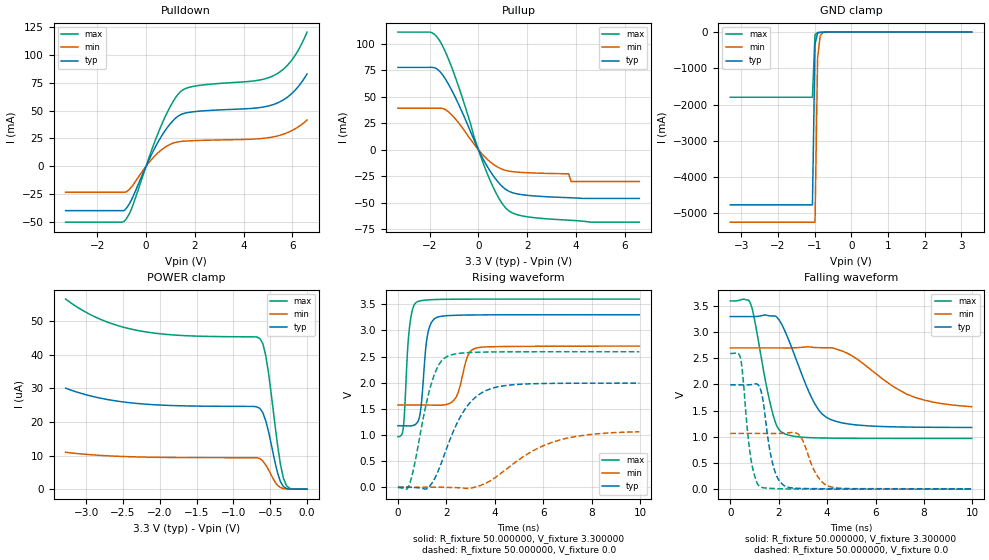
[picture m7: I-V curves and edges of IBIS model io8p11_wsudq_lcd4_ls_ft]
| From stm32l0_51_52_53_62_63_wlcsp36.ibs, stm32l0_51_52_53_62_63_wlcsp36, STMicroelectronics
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|   Model io8p11_wsudq_lcd4_ls_ft
[Model]  io8p11_wsudq_lcd4_ls_ft
Model_type I/O
Polarity   Non-Inverting
Enable   Active-Low
Vinl =   0.990000V
Vinh =   2.310000V
Vmeas =  1.650000V
Cref =   50.000000pF
Rref =   100.000000M
Vref =   0.0V
C_comp   3.263700pF   3.224800pF   3.309000pF
[Temperature Range]   25.000000   0.125000k   -40.000000
[Pullup Reference]   3.300000V   2.700000V   3.600000V
[Pulldown Reference]   0.0V   0.0V   0.0V
[POWER Clamp Reference]   3.300000V   2.700000V   3.600000V
[GND Clamp Reference]   0.0V   0.0V   0.0V
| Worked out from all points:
|   slope of the pulldown table from 0 to 0.495 V, typ, clamps not added: 22.6 ohm
|   slope of the pullup table from 0 to 0.495 V, typ, clamps not added: 23.9 ohm
|   GND clamp passes 1 mA (typ) near -0.64 V on its own axis
|   rising waveform, R_fixture 50.000000, V_fixture 3.300000: 20-80 % time 240ps typ, 378ps min, 202ps max; typ from 1.18 V to 3.3 V
|   rising waveform, R_fixture 50.000000, V_fixture 0.0: 20-80 % time 1.2ns typ, 2.22ns min, 722ps max; typ from 0 V to 1.99 V
|   falling waveform, R_fixture 50.000000, V_fixture 3.300000: 20-80 % time 1.14ns typ, 2.1ns min, 656ps max; typ from 3.3 V to 1.18 V
|   falling waveform, R_fixture 50.000000, V_fixture 0.0: 20-80 % time 417ps typ, 583ps min, 339ps max; typ from 1.99 V to 0 V
[Pulldown]
|Voltage   I(typ)   I(min)   I(max)
-3.3V     -39.83mA   -23.37mA   -50.2mA
-900mV    -39.83mA   -23.37mA   -49.52mA
-600mV    -30.28mA   -18.59mA   -38.45mA
500mV     22.11mA    12.28mA    30.1mA
1V        38.33mA    19.81mA    53.88mA
1.4V      46.1mA     22.18mA    66.72mA
2V        49.07mA    23.01mA    71.93mA
4.4V      52.05mA    24.38mA    76.53mA
5.2V      55.25mA    26.31mA    81.02mA
5.6V      59.18mA    28.57mA    86.57mA
6V        65.79mA    32.24mA    95.97mA
6.6V      82.83mA    41.41mA    120.4mA
[Pullup]
|Voltage   I(typ)   I(min)   I(max)
-3.3V     77.63mA    39.16mA    110.9mA
-2V       77.63mA    39.16mA    110.9mA
-1.6V     74.23mA    39.16mA    103.2mA
-1.3V     64.66mA    36.99mA    89.44mA
-900mV    47.13mA    27.82mA    65.37mA
300mV     -13.29mA   -7.65mA    -18.99mA
800mV     -30.32mA   -16.54mA   -44.19mA
1.2V      -38.62mA   -20mA      -56.79mA
1.9V      -42.8mA    -21.61mA   -62.92mA
3.7V      -45.29mA   -22.8mA    -66.5mA
3.8V      -45.39mA   -30mA      -66.64mA
6.6V      -46mA      -30mA      -68.41mA
[GND_clamp]
|Voltage   I(typ)   I(min)   I(max)
-3.3V     -4.767A    -5.245A    -1.798A
-1.06V    -4.767A    -5.245A    -1.798A
-990mV    -327.3mA   -5.245A    -68.38mA
-920mV    -29.22mA   -722.7mA   -11.24mA
-850mV    -6.771mA   -104.4mA   -6.721mA
-780mV    -3.56mA    -17.38mA   -4.326mA
-500mV    -59.41uA   -172uA     -34.91uA
3.28V     0A         0A         0A
[POWER_clamp]
|Voltage   I(typ)   I(min)   I(max)
-3.28V    30.09uA    10.99uA    56.63uA
-2.84V    27.27uA    10.11uA    50.92uA
-2.32V    25.55uA    9.609uA    47.36uA
-640mV    24.06uA    9.1uA      44.84uA
-600mV    22.76uA    8.366uA    43.37uA
-560mV    20.32uA    7.212uA    39.74uA
-520mV    16.86uA    5.676uA    34.15uA
-400mV    4.842uA    1.146uA    13.11uA
-360mV    2.185uA    478.4nA    7.29uA
-320mV    773nA      181.6nA    3.214uA
-240mV    60.58nA    0A         296.5nA
0V        0A         0A         0A
[Ramp]
| variable   typ   min   max
dV/dt_r  1.19406/1.19486n   0.60960/2.08655n   1.55532/0.71999n
dV/dt_f  1.27188/1.13237n   0.59190/1.86966n   1.57836/0.65485n
R_load = 50.000000
[Rising Waveform]
R_fixture= 50.000000
V_fixture= 3.300000
V_fixture_min= 2.700000
V_fixture_max= 3.600000
|time   V(typ)   V(min)   V(max)
0s        1.177V     1.573V     966.3mV
220.2ps   1.176V     1.573V     1.129V
460.5ps   1.173V     1.573V     2.986V
780.8ps   1.227V     1.574V     3.544V
940.9ps   1.484V     1.574V     3.568V
1.221ns   2.91V      1.572V     3.583V
1.582ns   3.244V     1.569V     3.591V
2.342ns   3.288V     1.682V     3.597V
3.183ns   3.296V     2.656V     3.599V
9.97ns    3.3V       2.7V       3.6V
[Rising Waveform]
R_fixture= 50.000000
V_fixture= 0.0
V_fixture_min= 0.0
V_fixture_max= 0.0
|time   V(typ)   V(min)   V(max)
0s        163.8uV    9.227uV    -5.568mV
360.4ps   32.05uV    -4.124uV   -37.18mV
480.5ps   -997.1uV   -7.779uV   64.92mV
1.361ns   49.43mV    176uV      1.953V
1.662ns   311.1mV    -250.6uV   2.319V
2.002ns   731.7mV    -2.637mV   2.494V
2.843ns   1.54V      -23.31mV   2.574V
3.804ns   1.88V      120.5mV    2.587V
6.366ns   1.986V     858.2mV    2.592V
9.97ns    1.992V     1.062V     2.592V
[Falling Waveform]
R_fixture= 50.000000
V_fixture= 3.300000
V_fixture_min= 2.700000
V_fixture_max= 3.600000
|time   V(typ)   V(min)   V(max)
0s        3.3V       2.7V       3.6V
860.9ps   3.299V     2.7V       3.519V
1.722ns   3.311V     2.7V       1.499V
1.922ns   3.288V     2.7V       1.207V
2.182ns   3.097V     2.7V       1.07V
3.343ns   1.763V     2.715V     980.1mV
4.024ns   1.356V     2.702V     972.3mV
5.005ns   1.236V     2.556V     968.5mV
7.287ns   1.184V     1.813V     966.7mV
9.97ns    1.177V     1.573V     966.3mV
[Falling Waveform]
R_fixture= 50.000000
V_fixture= 0.0
V_fixture_min= 0.0
V_fixture_max= 0.0
|time   V(typ)   V(min)   V(max)
0s        1.992V     1.062V     2.592V
420.4ps   1.992V     1.062V     2.508V
840.8ps   1.995V     1.062V     608.7mV
1.241ns   1.915V     1.062V     39.54mV
1.762ns   463.8mV    1.061V     7.24mV
2.302ns   42.98mV    1.069V     -330.9uV
2.883ns   9.462mV    1.01V      -3.155mV
3.483ns   4.372mV    335.6mV    -4.115mV
4.024ns   2.725mV    55.92mV    -4.594mV
9.97ns    163.8uV    9.227uV    -5.568mV
